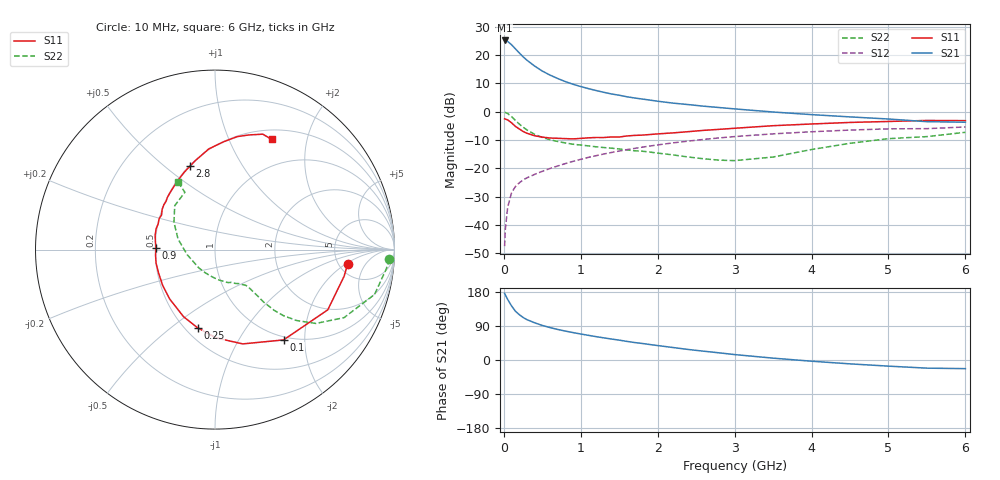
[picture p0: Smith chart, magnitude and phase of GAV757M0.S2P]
! Infineon Technologies  Discrete & RF Semiconductors
! BF775
! Si NPN RF Bipolar Junction Transistor in SOT23
! VCE = 0.75 V  IC = 7 mA
! Common Emitter S-Parameters:  May  1996
# GHz  S  MA  R  50
!  f  S11  S21  S12  S22
! GHz  MAG  ANG  MAG  ANG  MAG  ANG  MAG  ANG
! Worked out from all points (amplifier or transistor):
!   36 points, 10 MHz to 6 GHz, reference 50 ohm
!   highest |S21| = 25.1 dB at 10 MHz (marker M1)
!   |S21| within 3 dB of that: start of sweep to 151.8 MHz
!   unconditionally stable (mu >= 1): 560.7 MHz to end of sweep
!   at 250 MHz: K = 0.63, MSG = 21.8 dB, |S12| = -24.2 dB
!   at 1.4 GHz: K = 1.19, MAG = 7.7 dB, |S12| = -14.5 dB
!   at 6 GHz: K = 1.05, MAG = -0.6 dB, |S12| = -5.4 dB
!   S11 on the Smith chart (normalised r, x): 10 MHz: 6.06, -2.11; 100 MHz: 0.95, -1.58; 250 MHz: 0.57, -0.62; 900 MHz: 0.51, +0.01; 2.8 GHz: 0.51, +0.61; 6 GHz: 0.62, +1.45
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0.01  0.744 -6.0  17.97 175.9  0.0042 85.1  0.9736 -3.1
0.02  0.7347 -11.6  17.95 171.5  0.0085 83.9  0.9606 -6.4
0.05  0.7124 -28.1  17.27 159.7  0.0205 76.3  0.9234 -15.7
0.1  0.6318 -52.8  15.11 142.8  0.0367 66.2  0.8128 -27.8
0.15  0.5477 -73.6  12.8 128.9  0.0473 58.9  0.6967 -36.2
0.2  0.4924 -89.1  10.86 119.8  0.0551 55.4  0.6023 -41.0
0.25  0.446 -102.6  9.27 112.3  0.0618 53.7  0.5297 -44.0
0.3  0.4132 -115.0  8.063 106.5  0.0675 53.2  0.4741 -45.7
0.4  0.3736 -132.5  6.353 98.2  0.0777 53.3  0.3965 -47.2
0.5  0.3534 -145.6  5.177 91.2  0.088 54.2  0.3486 -47.4
0.6  0.3405 -157.2  4.398 85.6  0.0987 54.6  0.3185 -47.8
0.7  0.3369 -167.2  3.827 80.6  0.1093 55.5  0.2958 -48.0
0.9  0.3288 178.6  3.029 72.3  0.132 56.0  0.2646 -49.1
1.1  0.3434 166.1  2.537 65.1  0.1552 55.4  0.2474 -52.0
1.3  0.3474 155.9  2.183 58.4  0.1781 54.3  0.2313 -55.0
1.6  0.3706 142.5  1.822 49.1  0.2125 51.9  0.2102 -62.0
2.2  0.4198 123.0  1.407 32.9  0.2798 45.4  0.1715 -82.1
2.8  0.4849 106.7  1.176 18.9  0.3423 37.6  0.1386 -116.4
3.5  0.5623 93.5  0.981 4.9  0.4036 27.7  0.1573 -169.5
4.5  0.642 78.8  0.804 -10.2  0.4708 14.2  0.275 146.3
5.5  0.696 67.5  0.662 -21.5  0.4986 0.8  0.3608 117.7
6  0.6902 62.8  0.648 -22.8  0.5341 -3.1  0.4301 118.8
